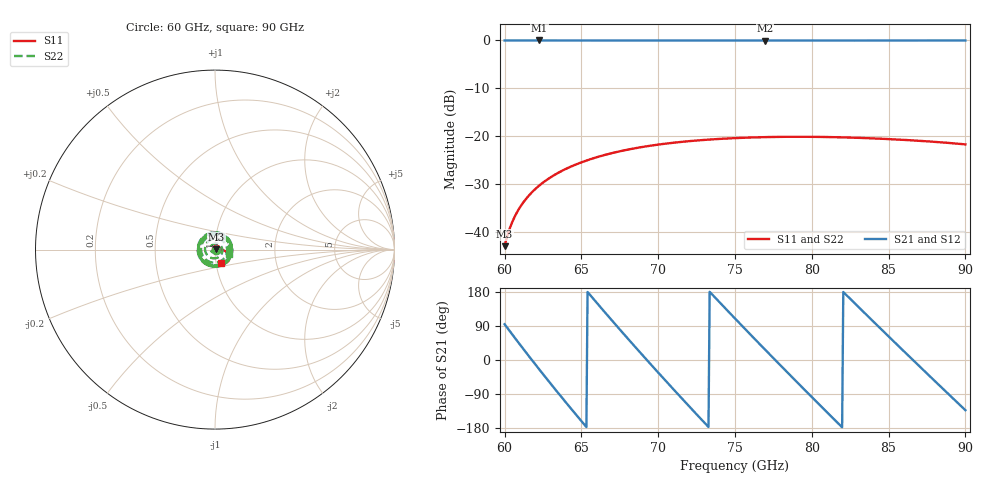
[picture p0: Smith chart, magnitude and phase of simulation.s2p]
! Touchstone file from project Project26
! Exported from HFSS 2014.0.7
! Variables:
!  wg2A = 122mil
!  wg2B = 61mil
!  wgA = 148mil
!  wgB = 74mil
!  wgLen = 1.616mm
!  wgLen2 = 122mil
!Data is not renormalized
# GHZ S MA
! Modal data exported
! Port[1] = 1:1
! Port[2] = 2:1
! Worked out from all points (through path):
!   401 points, 60 GHz to 90 GHz, reference per port
!   highest |S21| = -0.09 dB at 62.25 GHz (marker M1); lowest = -0.1 dB at 76.95 GHz (marker M2)
!   lowest |S11| = -43.0 dB at 60 GHz (marker M3), VSWR 1.01
!   |S11| at or under -10 dB: start of sweep to end of sweep
!   |S22| runs from -43.1 to -20.3 dB; largest |S21 - S12| = 1.8e-14
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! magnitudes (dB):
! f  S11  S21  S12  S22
! 60 GHz  -43.0  -0.1  -0.1  -43.1
! 60.08 GHz  -42.0  -0.1  -0.1  -42.1
! 60.3 GHz  -39.6  -0.1  -0.1  -39.7
! 60.45 GHz  -38.3  -0.1  -0.1  -38.5
! 60.67 GHz  -36.7  -0.1  -0.1  -36.9
! 60.9 GHz  -35.4  -0.1  -0.1  -35.6
! 61.2 GHz  -33.9  -0.1  -0.1  -34.1
! 61.5 GHz  -32.7  -0.1  -0.1  -32.9
! 62.25 GHz  -30.3  -0.1  -0.1  -30.5
! 62.85 GHz  -28.9  -0.1  -0.1  -29.1
! 63.45 GHz  -27.7  -0.1  -0.1  -27.9
! 64.2 GHz  -26.5  -0.1  -0.1  -26.7
! 65.03 GHz  -25.5  -0.1  -0.1  -25.6
! 66.08 GHz  -24.4  -0.1  -0.1  -24.5
! 67.28 GHz  -23.4  -0.1  -0.1  -23.5
! 70.05 GHz  -21.8  -0.1  -0.1  -21.9
! 72.38 GHz  -21.0  -0.1  -0.1  -21.1
! 75 GHz  -20.4  -0.1  -0.1  -20.6
! 76.95 GHz  -20.2  -0.1  -0.1  -20.4
! 80.03 GHz  -20.2  -0.1  -0.1  -20.3
! 85.05 GHz  -20.7  -0.1  -0.1  -20.8
! 90 GHz  -21.7  -0.1  -0.1  -21.9
